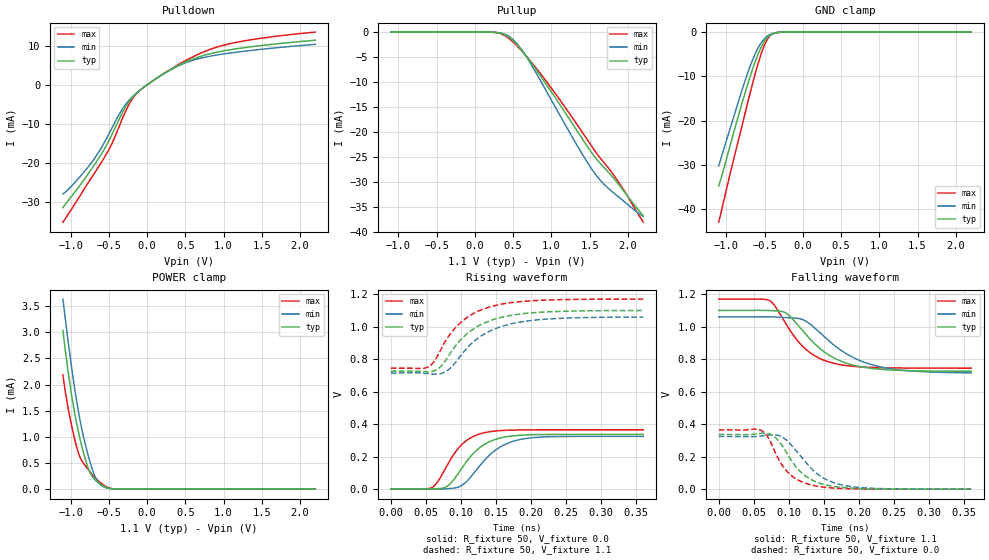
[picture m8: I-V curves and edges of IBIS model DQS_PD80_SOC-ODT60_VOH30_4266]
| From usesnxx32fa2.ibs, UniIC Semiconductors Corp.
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| DQS_PD80_SOC-ODT60_VOH30_4266
| (80 Ohm Pulldown, 60 Ohm System ODT Setting, VOH=VDDQ/3.0, 3200-4266Mbps)
[Model]   DQS_PD80_SOC-ODT60_VOH30_4266
Model_type   I/O
Vinl = 123.333mV
Vinh = 243.333mV
Vmeas = 183.333mV
Vref = 0.0mV
Cref = 0.0pF
Rref = 60.000Ohm
|   typ   min   max
|C_comp   0.849pF   0.799pF   0.899pF
C_comp_pullup   0.4245pF   0.3995pF   0.4495pF
C_comp_pulldown   0.4245pF   0.3995pF   0.4495pF
| Note: C_comp changes when the ODT circuit is enabled.
[Model Spec]
| Input threshold voltage corners
Vinl   0.1233V   0.1167V   0.1350V
Vinh   0.2433V   0.2367V   0.2550V
| Measurement voltage corners
Vmeas   0.1833V   0.1767V   0.1950V
| Timing spec test load voltage corners
Vref   0.0000V   0.0000V   0.0000V
| Dynamic Overshoot Parameters from LPDDR4 Specification
D_overshoot_ampl_h   0.30   NA   NA
D_overshoot_ampl_l   0.30   NA   NA
D_overshoot_area_h   0.1n   NA   NA
D_overshoot_area_l   0.1n   NA   NA
[Voltage Range]   1.1000V   1.0600V   1.1700V
[Pullup Reference]   1.1000V   1.0600V   1.1700V
| Junction Temperature (Ambient temp is 35C typ 95C min -40C max)
[Temperature Range]   50.0   110.0   -40.0
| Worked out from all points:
|   slope of the pulldown table from 0 to 0.165 V, typ, clamps not added: 74.2 ohm
|   slope of the pullup table from 0 to 0.165 V, typ, clamps not added: 19.5 kohm
|   GND clamp passes 1 mA (typ) near -0.45 V on its own axis
|   POWER clamp passes 1 mA (typ) near -0.88 V on its own axis
|   rising waveform, R_fixture 50, V_fixture 0.0: 20-80 % time 39.9ps typ, 44ps min, 34.9ps max; typ from 0.001 V to 0.337 V
|   falling waveform, R_fixture 50, V_fixture 1.1: 20-80 % time 57.8ps typ, 68.2ps min, 47.2ps max; typ from 1.1 V to 0.726 V
|   rising waveform, R_fixture 50, V_fixture 1.1: 20-80 % time 55.6ps typ, 57.7ps min, 52.2ps max; typ from 0.726 V to 1.1 V
|   falling waveform, R_fixture 50, V_fixture 0.0: 20-80 % time 38ps typ, 44.8ps min, 33.1ps max; typ from 0.337 V to 0.001 V
[Pulldown]
|   Voltage   I(typ)   I(min)   I(max)
-1.1V     -31.57mA   -28.05mA   -35.32mA
-760.1mV  -22.62mA   -20.87mA   -24.9mA
-624.8mV  -18.66mA   -17.07mA   -20.81mA
-512.6mV  -14.91mA   -13.17mA   -17.15mA
-334.4mV  -7.639mA   -6.616mA   -9.272mA
-209mV    -3.641mA   -3.404mA   -4.117mA
-139.7mV  -2.203mA   -2.144mA   -2.284mA
-40.7mV   -612.3uA   -606.3uA   -599.1uA
447.7mV   5.369mA    5.214mA    5.637mA
880mV     8.263mA    7.563mA    9.488mA
1.398V    9.879mA    8.934mA    11.71mA
2.2V      11.48mA    10.44mA    13.57mA
[GND Clamp]
|   Voltage   I(typ)   I(min)   I(max)
-1.1V     -34.74mA   -30.21mA   -42.91mA
-1.05V    -31.86mA   -27.33mA   -39.27mA
-941.6mV  -25.02mA   -21.26mA   -31.32mA
-796.4mV  -16.11mA   -13.14mA   -21.19mA
-664.4mV  -8.736mA   -6.578mA   -12.07mA
-588.5mV  -5.113mA   -3.681mA   -7.299mA
-519.2mV  -2.564mA   -1.832mA   -3.66mA
-466.4mV  -1.296mA   -941.8uA   -1.692mA
-413.6mV  -564.5uA   -418.4uA   -621.3uA
-354.2mV  -178.2uA   -135.3uA   -159.9uA
-258.5mV  -16.01uA   -14.34uA   -9.887uA
2.2V      0A         0A         0A
[Pullup]
|   Voltage   I(typ)   I(min)   I(max)
-1.1V     4.184uA    6.447uA    1.886uA
229.9mV   -30.19uA   -30.5uA    -31.03uA
338.8mV   -242.1uA   -199.7uA   -331.4uA
434.5mV   -925.6uA   -756.7uA   -1.171mA
553.3mV   -2.6mA     -2.398mA   -2.819mA
685.3mV   -5.106mA   -5.247mA   -5.061mA
1.075V    -13.71mA   -15.69mA   -12.83mA
1.411V    -21.57mA   -24.66mA   -20.25mA
1.566V    -25.01mA   -28.3mA    -23.76mA
1.695V    -27.27mA   -30.62mA   -26.29mA
1.87V     -30.35mA   -32.94mA   -29.89mA
2.2V      -36.89mA   -36.87mA   -38.1mA
[POWER Clamp]
|   Voltage   I(typ)   I(min)   I(max)
-1.1V     3.033mA    3.633mA    2.184mA
-1.041V   2.345mA    2.929mA    1.625mA
-977.9mV  1.723mA    2.241mA    1.16mA
-911.9mV  1.2mA      1.61mA     763.9uA
-852.5mV  818.2uA    1.148mA    543.6uA
-776.6mV  434.1uA    683.2uA    390.2uA
-713.9mV  239.3uA    373uA      278.6uA
-657.8mV  146.8uA    178.8uA    190.6uA
-595.1mV  80.78uA    68.28uA    109.2uA
-496.1mV  20.09uA    12.35uA    25.7uA
-390.5mV  2.037uA    1.393uA    1.77uA
2.2V      0A         0A         0A
[Ramp]
|   typ   min   max
| 20% - 80%
dV/dt_r   201.79m/39.95p   194.53m/44.01p   218.86m/34.95p
dV/dt_f   224.44m/57.74p   206.41m/68.16p   255.16m/47.10p
| 25% - 75%
|dV/dt_r   168.16m/31.83p   162.10m/35.09p   182.39m/27.83p
|dV/dt_f   187.04m/45.94p   172.01m/54.30p   212.63m/37.45p
R_load = 50
[Rising Waveform]
R_fixture = 50
V_fixture = 0.0
|   Time   V(typ)   V(min)   V(max)
0s        535.6uV    465.1uV    389.5uV
57ps      183.7uV    -5.999uV   6.857mV
66ps      2.126mV    -363.7uV   40.71mV
78ps      11.83mV    1.452mV    128.3mV
88ps      48.53mV    5.024mV    202.5mV
103ps     140.2mV    27.9mV     281.3mV
133ps     274mV      174.7mV    347mV
160ps     318.5mV    269.2mV    361.2mV
193ps     333.5mV    311.9mV    364.6mV
360ps     336.8mV    324.7mV    365.2mV
[Falling Waveform]
R_fixture   = 50
V_fixture   = 1.1
V_fixture_min = 1.06
V_fixture_max = 1.17
|   Time   V(typ)   V(min)   V(max)
0s        1.1V       1.06V      1.17V
72ps      1.099V     1.061V     1.162V
81ps      1.098V     1.059V     1.122V
95ps      1.086V     1.056V     1.024V
119ps     978.8mV    1.045V     882.2mV
139ps     886mV      983.9mV    815.6mV
163ps     811.1mV    891.5mV    775.8mV
197ps     758.5mV    799.7mV    754.2mV
235ps     736.6mV    749.1mV    747.3mV
360ps     725.9mV    716mV      744.7mV
[Rising Waveform]
R_fixture   = 50
V_fixture   = 1.1
V_fixture_min = 1.06
V_fixture_max = 1.17
|   Time   V(typ)   V(min)   V(max)
0s        725.5mV    714.2mV    744.7mV
53ps      721.7mV    710.8mV    751.7mV
62ps      728.1mV    707.8mV    787.1mV
75ps      773.5mV    716.3mV    889.5mV
89ps      862.5mV    763.4mV    978mV
106ps     946.4mV    855.2mV    1.048V
123ps     999.6mV    925mV      1.092V
142ps     1.037V     974.4mV    1.123V
210ps     1.088V     1.043V     1.162V
360ps     1.1V       1.059V     1.17V
[Falling Waveform]
R_fixture = 50
V_fixture = 0.0
|   Time   V(typ)   V(min)   V(max)
0s        336.9mV    324.8mV    365.2mV
57ps      341.9mV    326mV      367.6mV
75ps      335.7mV    334.9mV    281.3mV
87ps      289.2mV    328.2mV    170.8mV
99ps      209.5mV    292.4mV    102.1mV
115ps     114.2mV    213mV      52.27mV
133ps     56.57mV    123.7mV    24.86mV
158ps     21.72mV    50.05mV    9.081mV
193ps     6.087mV    14.09mV    2.476mV
360ps     626.3uV    611.6uV    417.2uV
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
